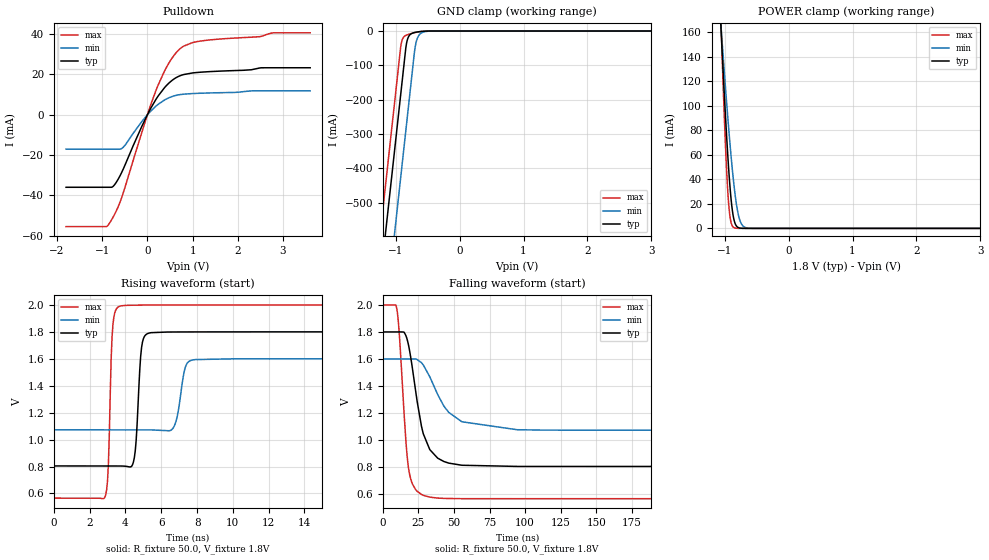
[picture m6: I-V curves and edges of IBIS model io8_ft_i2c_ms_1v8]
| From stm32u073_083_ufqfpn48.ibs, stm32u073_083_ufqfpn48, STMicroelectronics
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[Model]   io8_ft_i2c_ms_1v8
Model_type I/O_open_drain
Polarity   Non-Inverting
Enable   Active-Low
| CAP_THRESHOLD on pad IOFT is "UDTCAPC" :
| Rising=30.0% of vddiom   Falling=70.0% of vddiom
| C_comp min and max val. don't necessarily correlate with the min and max pvt
| but are the smallest and greatest pad capacitance found.
| var   typ   min   max
C_comp   2.35140pF  2.33125pF  2.40370pF
|C_comp_pulldown   2.35140pF  2.33125pF  2.40370pF
Vinl = 800.0mV
Vinh = 1.0V
Vmeas = 900.0mV   | Reference voltage for timing measurements
Cref  = 50.0pF   | Timing specification test load capacitance value
Rref  = 1.0MOhm   | Timing specification test load resistance value
Vref  = 990.0mV   | Timing specification test load voltage
[Model Spec]
| TIME_THRESHOLD on pin ZIV12 is "CMOS" :
| Rising=50.0% of vdd   Falling=50.0% of vdd
Vinl 728.70000mV 652.70000mV 817.70000mV
Vinh 1.06430V 953.30000mV 1.16330V
| variable   typ   min   max
[Temperature Range] 25.0 125.0 -40.0
| variable   typ   min   max
[Voltage Range] 1.8V 1.6V 2.0V
| variable   typ   min   max
[POWER Clamp Reference] 1.8V 1.6V 2.0V
| variable   typ   min   max
[GND Clamp Reference] 0V 0V 0V
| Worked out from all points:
|   slope of the pulldown table from 0 to 0.27 V, typ, clamps not added: 26.4 ohm
|   GND clamp passes 1 mA (typ) near -0.58 V on its own axis
|   POWER clamp passes 1 mA (typ) near -0.80 V on its own axis
|   rising waveform, R_fixture 50.0, V_fixture 1.8V: 20-80 % time 239ps typ, 365ps min, 181ps max; typ from 0.804 V to 1.8 V
|   falling waveform, R_fixture 50.0, V_fixture 1.8V: 20-80 % time 10.3ns typ, 18.2ns min, 5.33ns max; typ from 1.8 V to 0.804 V
[POWER Clamp]
-1.8V     1.076A     768.4mA    1.428A
-1.06V    166.8mA    167.3mA    172.4mA
-1.05V    156mA      159.9mA    156.7mA
-990mV    94.58mA    117mA      71.25mA
-950mV    58.69mA    90.08mA    29.27mA
-930mV    43.17mA    77.3mA     15.67mA
-910mV    29.83mA    65.11mA    7.377mA
-860mV    8.434mA    38.02mA    795.5uA
-810mV    1.577mA    17.81mA    74.4uA
-770mV    365.4uA    7.942mA    11.04uA
-650mV    4.138uA    347.7uA    35.9nA
3.6V      0A         0A         0A
[GND Clamp]
-1.8V     -1.68A     -1.921A    -1.54A
-1.24V    -727.6mA   -969.1mA   -588.3mA
-1.05V    -404.6mA   -646.1mA   -265.3mA
-920mV    -183.6mA   -425.1mA   -45.19mA
-890mV    -132.6mA   -374.1mA   -22.26mA
-850mV    -64.62mA   -306.1mA   -13.71mA
-830mV    -36.28mA   -272.1mA   -11.85mA
-800mV    -17.27mA   -221.1mA   -9.806mA
-690mV    -3.766mA   -41.92mA   -4.242mA
-640mV    -2.189mA   -13.56mA   -2.404mA
-570mV    -808.8uA   -3.218mA   -757.3uA
3.6V      453.9pA    48.38nA    315.2pA
| variable   typ   min   max
[Pullup Reference] 1.8V 1.6V 2.0V
| variable   typ   min   max
[Pulldown Reference] 0V 0V 0V
[Pulldown]
-1.8V     -35.95mA   -17.07mA   -55.42mA
-910mV    -35.95mA   -17.07mA   -55.42mA
-830mV    -35.95mA   -17.07mA   -53.41mA
-720mV    -34.49mA   -17.07mA   -49.08mA
-540mV    -27.18mA   -16.22mA   -39.07mA
-120mV    -5.598mA   -3.255mA   -8.496mA
240mV     9.353mA    5.171mA    14.85mA
490mV     15.96mA    8.523mA    26.14mA
750mV     19.54mA    10.04mA    33.17mA
1.37V     21.33mA    10.77mA    37.03mA
2.78V     23.25mA    11.81mA    40.55mA
3.6V      23.25mA    11.81mA    40.56mA
[Ramp]
dV/dt_r 597.43674mV/237.00156ps 316.63043mV/364.22789ps 860.76353mV/176.83325ps
dV/dt_f 597.4587mV/9.92807ns 316.65434mV/17.17546ns 860.78191mV/5.33364ns
R_load = 50.0
| Removed startup time: 0s 0s 0s  .
| Removed end time: 29.7ns.
[Rising Waveform]
R_fixture   = 50.0
V_fixture   = 1.8V
V_fixture_min = 1.6V
V_fixture_max = 2.0V
0s        804.2mV    1.072V     565.4mV
2.85ns    803.8mV    1.072V     571.3mV
3.05ns    803.8mV    1.072V     826.8mV
3.3ns     803.8mV    1.072V     1.851V
3.65ns    803.7mV    1.072V     1.989V
4.45ns    835.1mV    1.072V     1.998V
4.9ns     1.683V     1.072V     1.999V
5.3ns     1.79V      1.072V     1.999V
7.8ns     1.8V       1.592V     2V
29.7ns    1.8V       1.6V       2V
| Removed startup time: 0s 0s 0s  .
| Removed end time: 499.75ns.
[Falling Waveform]
R_fixture   = 50.0
V_fixture   = 1.8V
V_fixture_min = 1.6V
V_fixture_max = 2.0V
0s        1.8V       1.6V       2V
10.05ns   1.8V       1.6V       1.956V
16.68ns   1.759V     1.6V       928.5mV
19.55ns   1.615V     1.6V       712.8mV
27.13ns   1.102V     1.572V     596.9mV
33ns      928.5mV    1.468V     576.9mV
42.9ns    840.6mV    1.251V     567.6mV
55.53ns   813mV      1.135V     565.6mV
94.35ns   804.4mV    1.076V     565.4mV
499.8ns   804.2mV    1.072V     565.4mV
